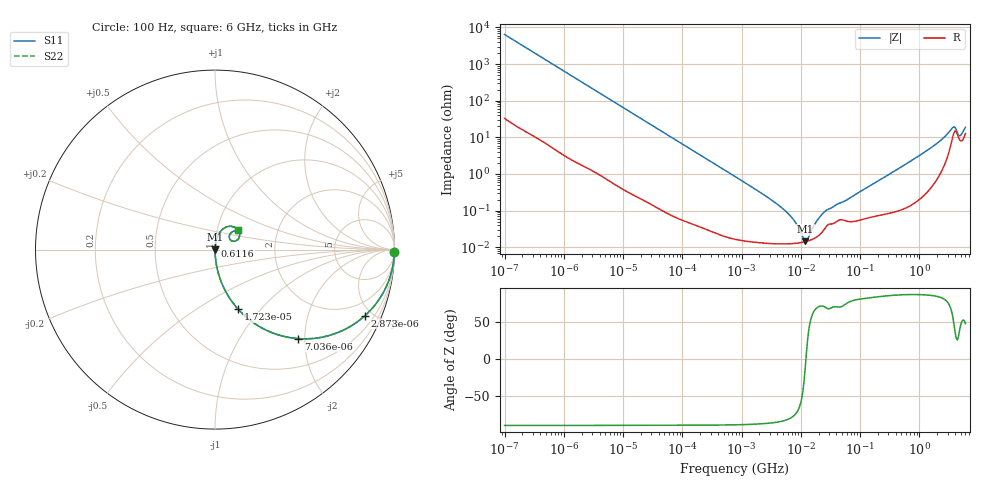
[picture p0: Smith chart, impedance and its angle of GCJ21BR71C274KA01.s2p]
!Murata Part Number: GCJ21BR71C274KA01
!These Parameters are Measured in Series Mode Connection
!Data Generated on Mar 13, 2026
!  o--ll--o
!Port1  Port2
!  o------o
!Operation Temp=25[degC], DC Bias Voltage=0[V]
!Freq. Start=100[Hz] Stop=6[GHz] 401[Steps]
# Hz S RI R 50
!Freq.(Hz) S11(Real) S11(Imag) S21(Real) S21(Imag) S12(Real) S12(Imag) S22(Real) S22(Imag)
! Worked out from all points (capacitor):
!   401 points, 100 Hz to 6 GHz, reference 50 ohm
!   read as one part in series: C = 247 nF near 109 Hz
!   lowest |Z| = 14.5 mohm at 11.89 MHz (marker M1)
!   series resonance near 12.21 MHz, so ESL is about 690 pH
!   S11 on the Smith chart (normalised r, x): 100 Hz: open; 2.873 kHz: 1.03, -4.53; 7.036 kHz: 1.01, -1.86; 17.23 kHz: 1.00, -0.76; 611.6 MHz: 1.00, +0.04; 6 GHz: 1.25, +0.28
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100  0.9997 -0.0155  0.00032 0.0155  0.00032 0.0155  0.9997 -0.0155
600  0.991 -0.0917  0.00896 0.0917  0.00896 0.0917  0.991 -0.0917
2008  0.9116 -0.2812  0.0884 0.2812  0.0884 0.2812  0.9116 -0.2812
2873  0.8354 -0.368  0.1646 0.368  0.1646 0.368  0.8354 -0.368
7036  0.463 -0.4958  0.537 0.4958  0.537 0.4958  0.463 -0.4958
17227  0.1278 -0.3308  0.8722 0.3308  0.8722 0.3308  0.1278 -0.3308
40335  0.0269 -0.1584  0.9731 0.1584  0.9731 0.1584  0.0269 -0.1584
774597  0.000239 -0.00856  0.9998 0.00856  0.9998 0.00856  0.000239 -0.00856
5311619  0.000125 -0.00102  0.9999 0.00102  0.9999 0.00102  0.000125 -0.00102
7947587  0.000128 -0.000488  0.9999 0.000488  0.9999 0.000488  0.000128 -0.000488
1.189169e7  0.000142 -2.92e-05  0.9999 2.92e-05  0.9999 2.92e-05  0.000142 -2.92e-05
1.300572e7  0.000148 7e-05  0.9999 -7e-05  0.9999 -7e-05  0.000148 7e-05
1.555665e7  0.000164 0.000272  0.9998 -0.000272  0.9998 -0.000272  0.000164 0.000272
2.035112e7  0.000214 0.0006  0.9998 -0.0006  0.9998 -0.0006  0.000214 0.0006
2.662322e7  0.000363 0.000937  0.9996 -0.000937  0.9996 -0.000937  0.000363 0.000937
3.124326e8  0.000941 0.00983  0.9991 -0.00983  0.9991 -0.00983  0.000941 0.00983
6.11557e8  0.00158 0.0192  0.9984 -0.0192  0.9984 -0.0192  0.00158 0.0192
1.873145e9  0.0101 0.0625  0.9899 -0.0625  0.9899 -0.0625  0.0101 0.0625
3.505958e9  0.0885 0.1302  0.9115 -0.1302  0.9115 -0.1302  0.0885 0.1302
3.8344e9  0.1297 0.1094  0.8703 -0.1094  0.8703 -0.1094  0.1297 0.1094
4.796499e9  0.0825 0.0577  0.9175 -0.0577  0.9175 -0.0577  0.0825 0.0577
6e9  0.1261 0.1073  0.8739 -0.1073  0.8739 -0.1073  0.1261 0.1073
